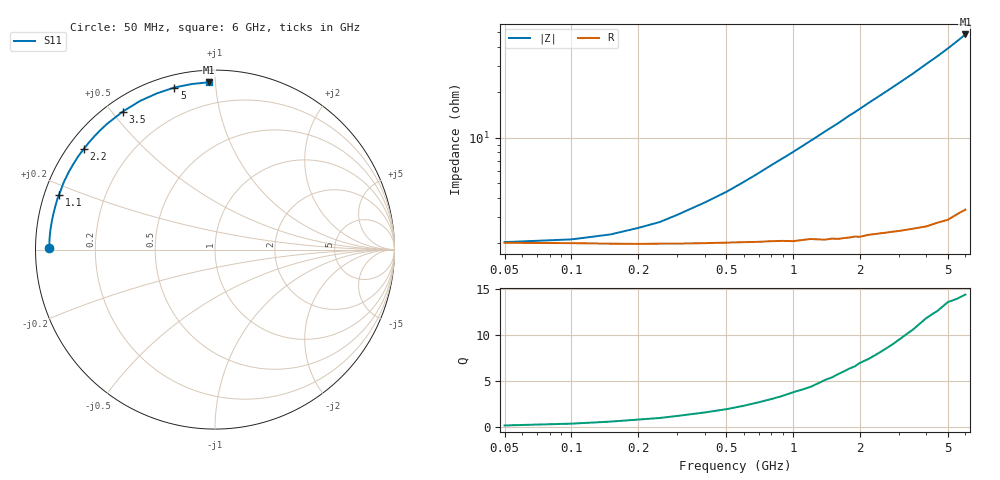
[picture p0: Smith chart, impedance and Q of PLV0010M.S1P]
! Infineon Technologies  Discrete & RF Semiconductors
! BAR 64-04W /-05W /-06W
! Si PIN Diode in SOT323
! IF = 10 mA
! S-Parameters:  October  2008
# GHz  S  MA  R  50
!  f  S11
! GHz  MAG  ANG
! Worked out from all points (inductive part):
!   34 points, 50 MHz to 6 GHz, reference 50 ohm
!   read as one part to ground: L = 1.24 nH near 800 MHz
!   highest Q = 14.4 at 6 GHz (marker M1), where L = 1.28 nH
!   S11 on the Smith chart (normalised r, x): 50 MHz: 0.04, +0.01; 1.1 GHz: 0.04, +0.17; 2.2 GHz: 0.05, +0.34; 3.5 GHz: 0.05, +0.53; 5 GHz: 0.06, +0.78; 6 GHz: 0.07, +0.96
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0.05  0.9226 179.3
0.1  0.9229 178.4
0.2  0.9238 176.4
0.25  0.9236 175.6
0.3  0.9236 174.6
0.4  0.9232 172.8
0.5  0.9228 171.1
0.6  0.9224 169.3
0.7  0.9223 167.5
0.8  0.9218 165.7
1  0.9224 162.3
1.1  0.9215 160.6
1.4  0.9223 155.5
1.6  0.9224 152.3
1.8  0.922 148.9
1.9  0.9215 147.4
2  0.9224 145.8
2.2  0.9214 142.6
2.4  0.9217 139.6
2.6  0.922 136.6
2.8  0.9225 133.7
3  0.9233 130.8
3.5  0.925 123.8
4  0.9275 116.8
4.5  0.9286 110.4
5  0.9312 104.1
5.5  0.9315 97.9
6  0.9331 92.0
